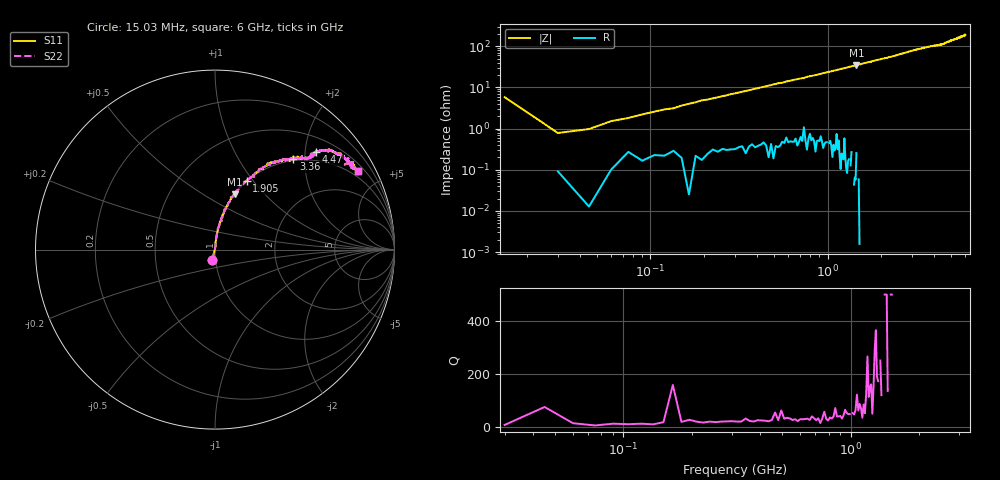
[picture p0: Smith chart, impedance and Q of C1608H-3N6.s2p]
!	Network	Analyzer	HP8753E.07.74:	Oct	30	2002	Serial	No.	JP38451487
!	Hewlett-Packard
!	7	Sep	2009	10:11:20
!	Frequency	S11	S21	S12	S22
#	HZ	S	RI	R	50
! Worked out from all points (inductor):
!   400 points, 15.03 MHz to 6 GHz, reference 50 ohm
!   read as one part in series: L = 3.8 nH near 45.03 MHz
!   highest Q = 521 at 1.455 GHz (marker M1), where L = 3.79 nH
!   S11 on the Smith chart (normalised r, x): 15.03 MHz: 0.96, -0.11; 1.905 GHz: 1.00, +0.93; 3.36 GHz: 0.97, +1.77; 4.47 GHz: 0.80, +2.24; 6 GHz: 0.76, +3.75
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1.502992e7  -0.0152 -0.0565  1.02 0.0565  1.02 0.0565  -0.0152 -0.0565
3.002985e7  0.000947 0.00776  0.999 -0.00776  0.999 -0.00776  0.000947 0.00776
4.502978e7  0.000446 0.00975  1 -0.00975  1 -0.00975  0.000446 0.00975
6.00297e7  0.00147 0.0151  0.999 -0.0151  0.999 -0.0151  0.00147 0.0151
1.200294e8  0.00308 0.029  0.997 -0.029  0.997 -0.029  0.00308 0.029
1.95029e8  0.00413 0.0482  0.996 -0.0482  0.996 -0.0482  0.00413 0.0482
2.850286e8  0.00761 0.0682  0.992 -0.0682  0.992 -0.0682  0.00761 0.0682
5.250274e8  0.0189 0.123  0.981 -0.123  0.981 -0.123  0.0189 0.123
1.020025e9  0.0575 0.224  0.942 -0.224  0.942 -0.224  0.0575 0.224
1.455023e9  0.109 0.308  0.891 -0.308  0.891 -0.308  0.109 0.308
1.90502e9  0.177 0.381  0.823 -0.381  0.823 -0.381  0.177 0.381
2.01002e9  0.193 0.395  0.807 -0.395  0.807 -0.395  0.193 0.395
3.015015e9  0.378 0.506  0.622 -0.506  0.622 -0.506  0.378 0.506
3.360013e9  0.437 0.505  0.563 -0.505  0.563 -0.505  0.437 0.505
4.00501e9  0.523 0.515  0.477 -0.515  0.477 -0.515  0.523 0.515
4.470008e9  0.565 0.543  0.435 -0.543  0.435 -0.543  0.565 0.543
5.010005e9  0.678 0.535  0.322 -0.535  0.322 -0.535  0.678 0.535
5.355003e9  0.744 0.508  0.256 -0.508  0.256 -0.508  0.744 0.508
5.535002e9  0.72 0.474  0.28 -0.474  0.28 -0.474  0.72 0.474
5.565002e9  0.77 0.489  0.23 -0.489  0.23 -0.489  0.77 0.489
5.595002e9  0.737 0.481  0.263 -0.481  0.263 -0.481  0.737 0.481
6e9  0.795 0.437  0.205 -0.437  0.205 -0.437  0.795 0.437
